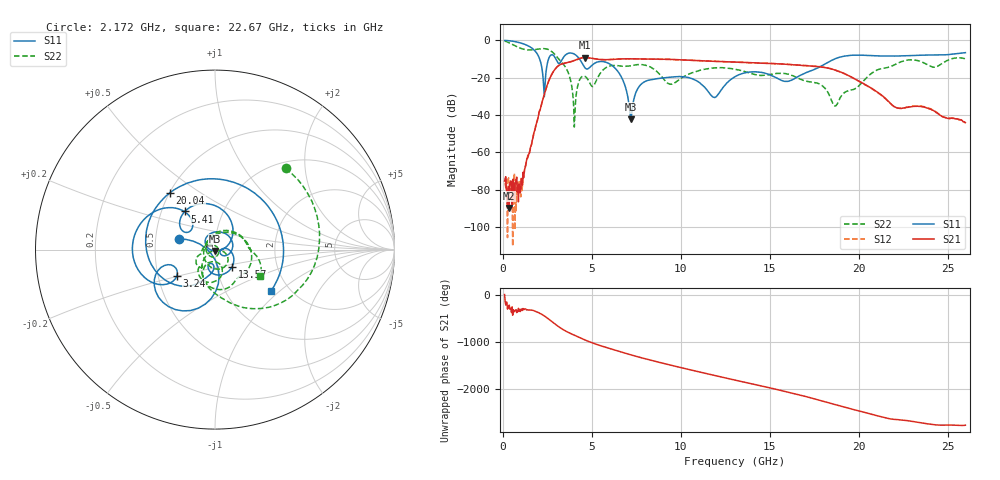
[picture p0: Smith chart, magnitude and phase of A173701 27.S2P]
!  2-Port S-parameters saved by WinCal
! VAR MeasName=S-Parameters (CALIBRATED_DATA) read from VNA (N5245A)
! VAR MeasDate=2017-6-7 10:30:10
! VAR NAME=A173701 27
! VAR FILENAME=A173701 27.S2P
! VAR DATE=2017-6-7 10:30:10
! VAR PHYS_PORTS=1,2
# Hz S DB R 50
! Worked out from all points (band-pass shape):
!   801 points, 100 MHz to 26 GHz, reference 50 ohm
!   highest |S21| = -9.18 dB at 4.633 GHz (marker M1); lowest = -89.7 dB at 359 MHz (marker M2)
!   |S21| within 3 dB of the highest: 3.489 GHz to 14.6 GHz (11.11 GHz wide, 123 % of centre); 14.61413 GHz to 14.66229 GHz (48.16 MHz wide, 0.329 % of centre)
!   lowest |S11| = -42.3 dB at 7.19 GHz (marker M3), VSWR 1.02, Z = 50 - j0.77 ohm
!   |S11| at or under -10 dB: 2.072 GHz to 2.569 GHz (496.9 MHz wide, 21.4 % of centre); 2.983 GHz to 3.343 GHz (360.8 MHz wide, 11.4 % of centre); 4.314 GHz to 18.64 GHz (14.32 GHz wide, 125 % of centre)
!   |S22| runs from -46.4 to -0.3 dB; largest |S21 - S12| = 0.0041
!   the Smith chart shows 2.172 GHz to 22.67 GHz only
!   S11 on the Smith chart (normalised r, x): 2.172 GHz: 0.66, +0.08; 3.24 GHz: 0.62, -0.20; 5.41 GHz: 0.66, +0.30; 13.57 GHz: 1.19, -0.23; 20.04 GHz: 0.50, +0.38; 22.67 GHz: 1.61, -0.88
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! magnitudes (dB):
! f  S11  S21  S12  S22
! 100 MHz  0.0  -75.3  -76.5  -0.3
! 359 MHz  -0.2  -89.7  -74.9  -1.3
! 1.006 GHz  -1.4  -79.0  -83.8  -4.2
! 2.172 GHz  -13.6  -34.2  -34.2  -4.4
! 3.24 GHz  -11.7  -12.9  -12.9  -11.0
! 4.017 GHz  -7.3  -10.7  -10.7  -46.4
! 4.438 GHz  -11.9  -9.4  -9.4  -19.4
! 4.633 GHz  -14.8  -9.2  -9.2  -19.4
! 5.41 GHz  -11.3  -10.2  -10.2  -18.6
! 6.543 GHz  -17.6  -10.0  -10.0  -13.6
! 7.19 GHz  -42.3  -9.8  -9.8  -13.6
! 7.74 GHz  -23.8  -9.9  -9.9  -12.9
! 8.744 GHz  -20.4  -10.0  -10.1  -17.5
! 11.88 GHz  -30.6  -11.2  -11.2  -14.7
! 13.05 GHz  -19.4  -11.6  -11.6  -15.4
! 13.57 GHz  -17.4  -11.8  -11.8  -16.6
! 17.39 GHz  -16.0  -13.8  -13.7  -22.4
! 18.68 GHz  -9.8  -15.9  -15.9  -35.0
! 20.04 GHz  -7.9  -21.9  -22.0  -24.0
! 21.69 GHz  -8.4  -32.8  -33.0  -14.3
! 22.67 GHz  -8.2  -35.9  -35.8  -10.7
! 26 GHz  -6.5  -44.0  -44.0  -9.9
